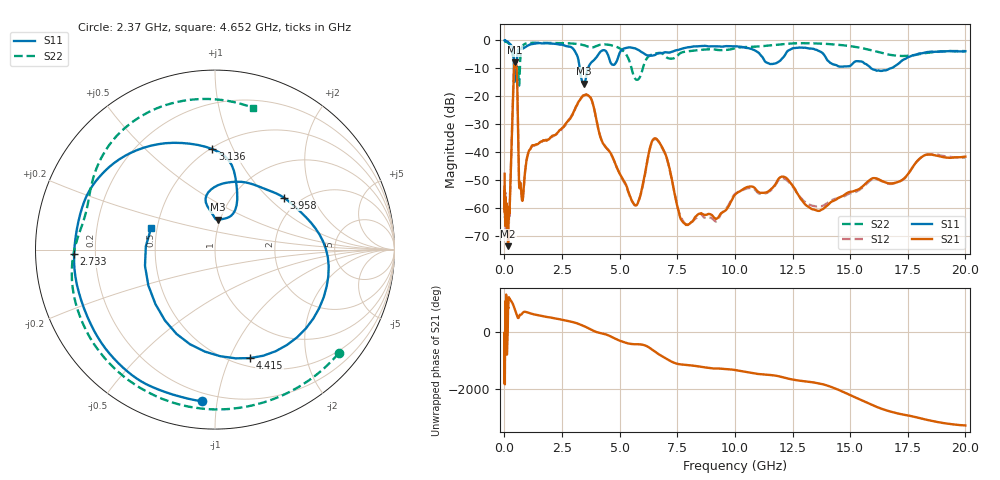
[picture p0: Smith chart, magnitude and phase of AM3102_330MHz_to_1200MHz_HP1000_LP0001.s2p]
! Date/Time: Tue, Sep 11, 2018 5:16 PM
! Network Analyzer: Agilent Technologies E8362B Rev: A.07.50.63
! Sweep from 0.010 to 20.000 GHz, 1601 Points, Sweep Type: LOG
! Power Supply: 4.949 V, 0.001 A
# Hz S DB R 50
!freq MagS11 AngS11 MagS21 AngS21 MagS12 AngS12 MagS22 AngS22
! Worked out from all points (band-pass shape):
!   1601 points, 10 MHz to 20 GHz, reference 50 ohm
!   highest |S21| = -7.87 dB at 455.8 MHz (marker M1); lowest = -73.8 dB at 158 MHz (marker M2)
!   |S21| within 3 dB of the highest: 410.8 MHz to 536.1 MHz (125.2 MHz wide, 26.5 % of centre)
!   lowest |S11| = -15.6 dB at 3.449 GHz (marker M3), VSWR 1.40, Z = 48.7 + j16.6 ohm
!   |S11| at or under -10 dB: 416.9 MHz to 464 MHz (47.11 MHz wide, 10.7 % of centre); 3.268 GHz to 3.628 GHz (359.9 MHz wide, 10.4 % of centre); 15.91 GHz to 16.76 GHz (845.9 MHz wide, 5.18 % of centre)
!   |S22| runs from -16.2 to -0.2 dB; largest |S21 - S12| = 0.0059
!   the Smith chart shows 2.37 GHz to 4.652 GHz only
!   S11 on the Smith chart (normalised r, x): 2.37 GHz: 0.15, -0.91; 2.733 GHz: 0.12, -0.02; 3.136 GHz: 0.51, +0.83; 3.958 GHz: 1.66, +1.25; 4.415 GHz: 0.59, -1.19; 4.652 GHz: 0.46, +0.13
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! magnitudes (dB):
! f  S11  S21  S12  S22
! 10 MHz  0.0  -47.8  -53.3  -0.2
! 35.55 MHz  0.0  -64.4  -63.0  -0.3
! 126.4 MHz  -0.4  -64.7  -63.0  -0.7
! 158 MHz  -0.5  -73.8  -68.1  -0.9
! 252.9 MHz  -1.2  -54.7  -54.3  -1.7
! 447.2 MHz  -14.3  -7.9  -8.0  -6.4
! 455.8 MHz  -12.3  -7.9  -7.9  -6.4
! 535.7 MHz  -7.6  -10.8  -10.8  -12.1
! 638.6 MHz  -3.1  -51.5  -51.6  -16.2
! 768.6 MHz  -2.9  -57.3  -57.5  -2.3
! 1.59 GHz  -1.0  -36.3  -36.2  -0.8
! 2.37 GHz  -1.4  -32.4  -32.9  -0.9
! 2.733 GHz  -2.1  -29.1  -29.5  -1.0
! 3.136 GHz  -5.0  -23.4  -23.4  -1.2
! 3.449 GHz  -15.6  -19.7  -19.7  -1.7
! 3.958 GHz  -6.4  -27.1  -27.0  -2.1
! 4.415 GHz  -3.9  -38.5  -38.4  -1.4
! 4.652 GHz  -8.5  -41.1  -41.2  -1.8
! 5.652 GHz  -2.8  -59.1  -59.0  -13.5
! 6.549 GHz  -5.1  -35.1  -35.3  -4.7
! 7.92 GHz  -2.5  -66.0  -65.9  -3.9
! 20 GHz  -3.9  -41.7  -42.0  -3.8
